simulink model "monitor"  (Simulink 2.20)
settings: Solver=ode45  StartTime=0.0  StopTime=10.0  RelTol=1e-3  AbsTol=1e-6
libraries: simulink x1

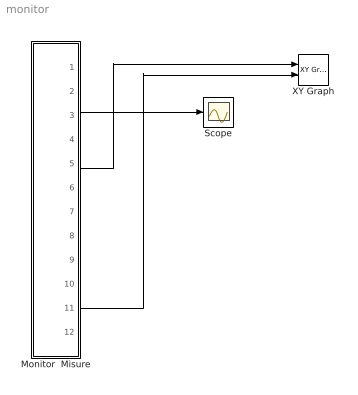
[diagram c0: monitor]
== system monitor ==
  Monitor  Misure : Subsystem
  Scope : Scope
  XY Graph : simulink/Sinks/XY Graph  xmin=-50  xmax=50  ymin=-50  ymax=50  st=-1
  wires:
  Monitor  Misure/3(x3) -> Scope/1
  Monitor  Misure/5(x5) -> XY Graph/1
  Monitor  Misure/11(y5) -> XY Graph/2

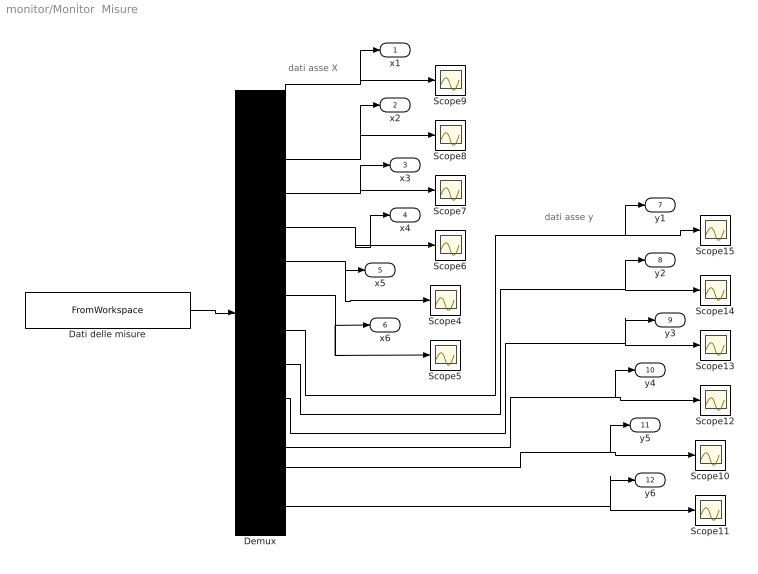
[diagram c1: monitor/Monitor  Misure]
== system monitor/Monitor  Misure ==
  note: dati asse y
  note: dati asse X
  Dati delle misure : FromWorkspace  VariableName=out
  Demux : Demux  Outputs=12
  Scope{4..15} (12 alike) : Scope
  x1 : Outport  Port=1
  x2 : Outport  Port=2
  x3 : Outport  Port=3
  x4 : Outport  Port=4
  x5 : Outport  Port=5
  x6 : Outport  Port=6
  y1 : Outport  Port=7
  y2 : Outport  Port=8
  y3 : Outport  Port=9
  y4 : Outport  Port=10
  y5 : Outport  Port=11
  y6 : Outport  Port=12
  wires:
  Dati delle misure/1 -> Demux/1
  Demux/1 -> Scope9/1, x1/1
  Demux/2 -> Scope8/1, x2/1
  Demux/3 -> Scope7/1, x3/1
  Demux/4 -> Scope6/1, x4/1
  Demux/5 -> Scope4/1, x5/1
  Demux/6 -> Scope5/1, x6/1
  Demux/12 -> Scope11/1, y6/1
  Demux/11 -> Scope10/1, y5/1
  Demux/10 -> Scope12/1, y4/1
  Demux/9 -> Scope13/1, y3/1
  Demux/8 -> Scope14/1, y2/1
  Demux/7 -> Scope15/1, y1/1
